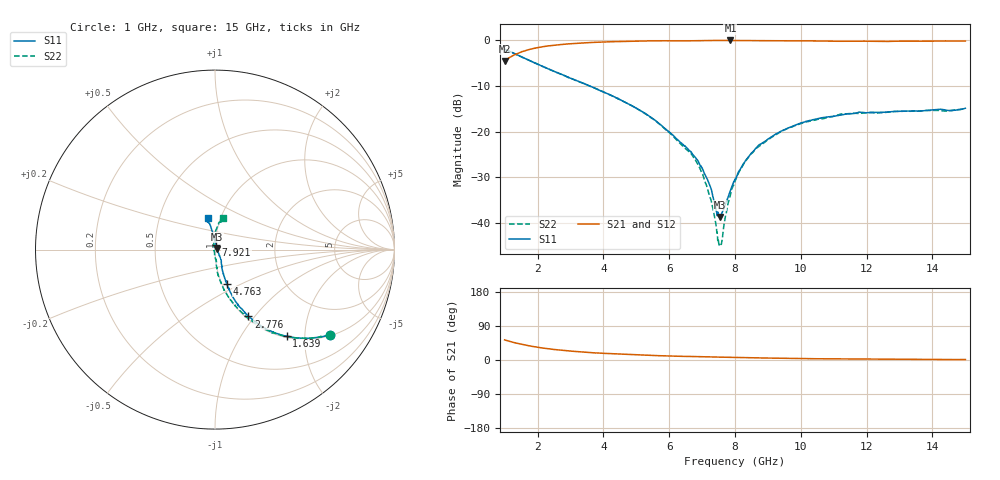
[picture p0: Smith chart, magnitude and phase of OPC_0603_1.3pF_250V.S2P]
! FILE NAME
! DATE 08/21/2012  10:37
! CORRECTED  DATA
# GHz  S  MA  R  50.00
!  FREQ  S11M  S11A  S21M  S21A  S12M  S12A  S22M  S22A
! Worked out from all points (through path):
!   1601 points, 1 GHz to 15 GHz, reference 50 ohm
!   highest |S21| = -0.06 dB at 7.86 GHz (marker M1); lowest = -4.5 dB at 1 GHz (marker M2)
!   group delay of S21, straight-line fit = 6.98 ps
!   lowest |S11| = -38.6 dB at 7.554 GHz (marker M3), VSWR 1.02, Z = 51.1 + j0.357 ohm
!   |S11| at or under -10 dB: 3.583 GHz to end of sweep
!   |S22| runs from -45.0 to -2.0 dB; largest |S21 - S12| = 0.0089
!   S11 on the Smith chart (normalised r, x): 1 GHz: 1.03, -2.68; 1.639 GHz: 1.03, -1.63; 2.776 GHz: 1.03, -0.93; 4.763 GHz: 1.05, -0.42; 7.921 GHz: 1.01, +0.05; 15 GHz: 0.87, +0.32
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1  0.7973 -36.5  0.5933 53.2  0.593 53.0  0.7974 -36.5
1.63875  0.6264 -50.3  0.769 39.3  0.7689 39.1  0.6267 -50.5
2.77625  0.4165 -63.4  0.9014 25.4  0.9006 25.4  0.4158 -64.8
3.33625  0.3449 -66.9  0.9309 21.3  0.93 21.3  0.3438 -69.3
4.7625  0.2008 -71.1  0.9729 14.5  0.9727 14.4  0.2007 -79.0
5.6725  0.1246 -70.5  0.9849 11.4  0.9845 11.4  0.1235 -84.2
6.62625  0.06144 -57.5  0.9835 9.3  0.9831 9.3  0.05866 -83.7
6.87125  0.04826 -55.4  0.9876 8.9  0.9869 8.9  0.04423 -88.9
7.23  0.02621 -43.1  0.9905 8.2  0.99 8.2  0.01973 -96.2
7.43125  0.0136 -20.7  0.9916 7.7  0.9908 7.7  0.00885 -116.8
7.50125  0.01246 1.7  0.9914 7.7  0.9907 7.6  0.006164 -138.9
7.55375  0.01169 17.4  0.992 7.6  0.9908 7.5  0.005759 -177.9
7.86  0.02288 73.0  0.9929 7.0  0.9917 6.9  0.02036 110.3
7.92125  0.02592 77.5  0.9922 6.8  0.992 6.8  0.02461 105.3
8  0.03024 81.5  0.9924 6.7  0.9912 6.7  0.02862 104.3
8.30625  0.04729 91.3  0.9911 6.2  0.9903 6.1  0.04683 97.0
8.6825  0.06889 95.3  0.9898 5.7  0.9892 5.6  0.06707 92.2
9.49625  0.105 98.6  0.9868 4.5  0.9865 4.5  0.1044 87.6
10.33625  0.1341 100.5  0.9825 3.5  0.9815 3.4  0.1316 83.0
11.24625  0.1524 103.3  0.9733 2.8  0.9727 2.8  0.1564 80.2
12.6725  0.1642 106.6  0.9694 2.2  0.9692 2.1  0.1636 77.4
15  0.1802 102.3  0.9795 1.3  0.9788 1.3  0.1791 75.6
